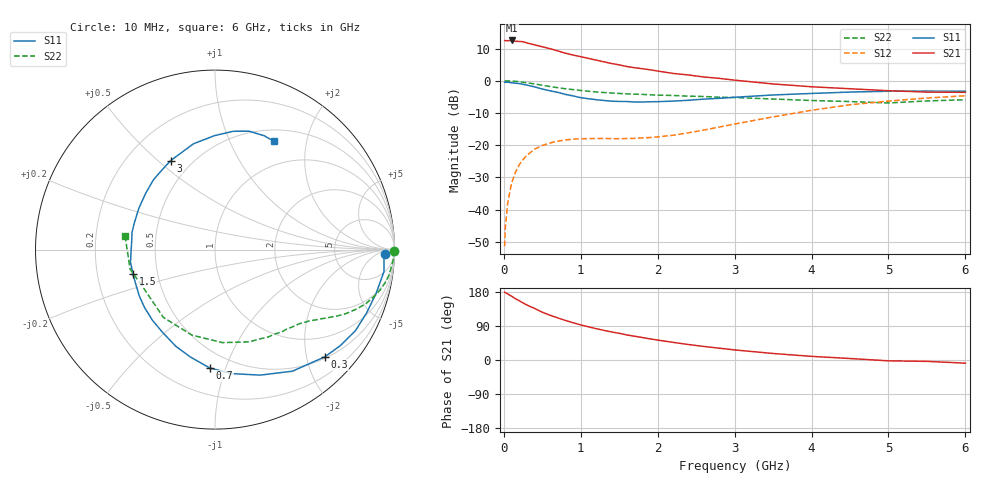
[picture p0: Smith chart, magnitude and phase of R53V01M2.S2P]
! SIEMENS Small Signal Semiconductors
! BFR183
! Si NPN RF Bipolar Junction Transistor in SOT23
! VCE = 3 V  IC = 1.2 mA
! Common Emitter S-Parameters:  May  1996
# GHz  S  MA  R  50
!  f  S11  S21  S12  S22
! GHz  MAG  ANG  MAG  ANG  MAG  ANG  MAG  ANG
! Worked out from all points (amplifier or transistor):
!   36 points, 10 MHz to 6 GHz, reference 50 ohm
!   highest |S21| = 12.5 dB at 100 MHz (marker M1)
!   |S21| within 3 dB of that: start of sweep to 665.1 MHz
!   unconditionally stable (mu >= 1): 1.574 GHz to 2.91 GHz
!   at 250 MHz: K = 0.17, MSG = 18.3 dB, |S12| = -24.5 dB
!   at 1.4 GHz: K = 0.91, MSG = 11.7 dB, |S12| = -18.0 dB
!   at 6 GHz: K = 0.94, MSG = 0.5 dB, |S12| = -4.7 dB
!   S11 on the Smith chart (normalised r, x): 10 MHz: 29, -14; 300 MHz: 0.53, -2.36; 700 MHz: 0.38, -0.88; 1.5 GHz: 0.36, -0.13; 3 GHz: 0.38, +0.55; 6 GHz: 0.65, +1.48
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0.01  0.946 -1.5  4.22 179.2  0.0027 87.0  0.9974 -0.5
0.02  0.9431 -3.0  4.189 177.6  0.0054 89.7  0.9907 -1.1
0.05  0.9494 -7.4  4.184 174.2  0.0125 84.4  0.9962 -2.8
0.1  0.9301 -15.2  4.221 168.5  0.0256 80.7  0.9869 -5.7
0.15  0.9153 -22.7  4.097 161.9  0.0376 76.1  0.9795 -8.5
0.25  0.8796 -37.5  4.034 150.5  0.0599 68.1  0.9481 -13.6
0.3  0.8552 -44.3  3.864 145.1  0.0697 64.8  0.929 -15.9
0.4  0.8032 -57.5  3.609 136.0  0.0866 57.8  0.8923 -19.8
0.5  0.7433 -70.2  3.371 126.1  0.0988 52.2  0.8508 -23.1
0.6  0.6978 -82.1  3.148 118.2  0.108 47.0  0.8125 -26.0
0.7  0.6605 -92.5  2.906 111.1  0.1152 43.3  0.7795 -28.2
0.9  0.581 -112.1  2.501 98.3  0.1241 37.4  0.7279 -31.6
1.1  0.5256 -131.6  2.223 87.6  0.1264 34.5  0.6869 -34.7
1.3  0.4943 -148.7  1.967 78.3  0.1271 33.7  0.6566 -37.3
1.5  0.4771 -163.5  1.763 70.4  0.126 34.8  0.6345 -40.0
1.9  0.4721 168.3  1.48 55.8  0.1312 41.2  0.6056 -45.9
2.2  0.4828 151.5  1.299 46.6  0.1423 47.1  0.5906 -50.9
3  0.5537 116.6  1.021 26.6  0.2126 56.1  0.5489 -69.5
3.5  0.6013 101.6  0.891 17.2  0.2747 54.2  0.5199 -85.4
4.5  0.6672 81.2  0.751 3.9  0.4237 41.5  0.4749 -127.3
5.5  0.6909 66.7  0.666 -3.6  0.539 25.1  0.4854 -167.0
6  0.6873 61.3  0.661 -8.3  0.5848 15.2  0.5069 171.3
